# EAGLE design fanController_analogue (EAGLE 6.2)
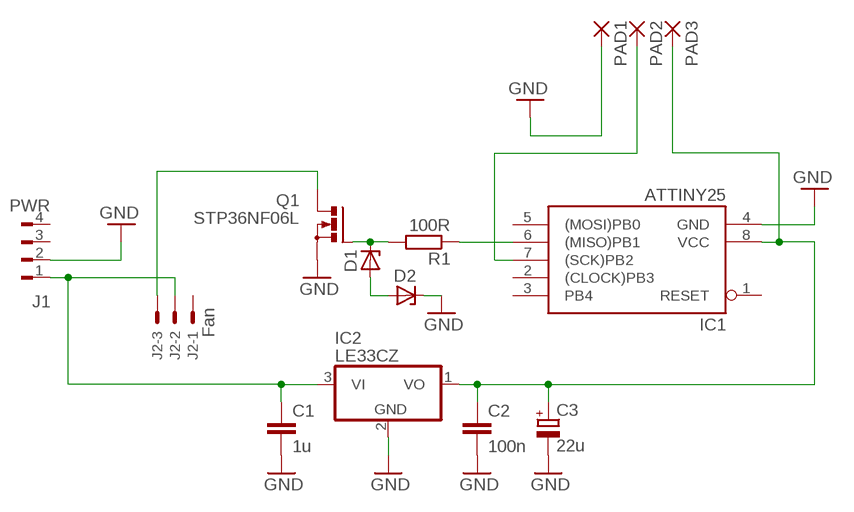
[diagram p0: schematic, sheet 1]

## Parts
C1  1u  C2.5/2  [C2.5-2]
C2  100n  C2.5/2  [C2.5-2]
C3  22u  CPOL-EUE2-4  [E2-4]
D1  ZENER-DIODEZD-5  [ZDIO-5]
D2  ZENER-DIODEZD-5  [ZDIO-5]
IC1  ATTINY25  TINY22P  [DIL08]
IC2  LE33CZ  78L05Z  [TO92]
J1  PWR  FLOP-4W827001  [827001]
J2  Fan  22-23-2031  [22-23-2031]
PAD1  2,54/1,1  [2,54/1,1]
PAD2  2,54/1,1  [2,54/1,1]
PAD3  2,54/1,1  [2,54/1,1]
Q1  STP36NF06L  BUZ11BV  [TO220BV]
R1  100R  R-EU_0207/7  [0207/7]

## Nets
GND: C1.2 C2.2 C3.- D2.C IC1.4(GND) IC2.2(GND) J1.2 PAD1.1(P) Q1.S
N$1: D1.C Q1.G R1.2
N$2: C1.1 IC2.3(VI) J1.1 J2.2
N$3: IC1.7((SCK)PB2) PAD2.1(P)
N$5: D1.A D2.A
N$6: IC1.6((MISO)PB1) R1.1
N$9: J2.3 Q1.D
VCC: C2.1 C3.+ IC1.8(VCC) IC2.1(VO) PAD3.1(P)
Unconnected: IC1.1(RESET) IC1.2((CLOCK)PB3) IC1.3(PB4) IC1.5((MOSI)PB0) J1.3 J1.4 J2.1

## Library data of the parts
C1 C2 = capacitor-wima:C: CAPACITOR
C3 = rcl:CPOL-EU: POLARIZED CAPACITOR, European symbol
D1 D2 = diode:ZENER-DIODE: Z-Diode
IC1 = atmel:TINY22: MICROCONTROLLER 1K ROM 128 bytes RAM 128 bytes EEPROM; OC_FARNELL: unknown; OC_NEWARK: unknown
IC2 = linear:78*: Positive VOLTAGE REGULATOR Source: http://cache.national.com/ds/LM/LM78L05.pdf http://www.fairchildsemi.com/ds/LM/LM7805.pdf
J1 = con-amp:FLOP-4W: MATE N-LOCK Floppy / HDD conector Distributor: Bürklin 71F972
J2 = con-molex:22-23-2031: .100" (2.54mm) Center Header - 3 Pin; MF: MOLEX; MPN: 22-23-2031; OC_FARNELL: 1462950; OC_NEWARK: 30C0862
PAD1-PAD3 = wirepad:2,54/1,1: THROUGH-HOLE PAD
Q1 = transistor-power:BUZ11: N-CHANNEL MOS FET
R1 = resistor:R-EU_: RESISTOR, European symbol

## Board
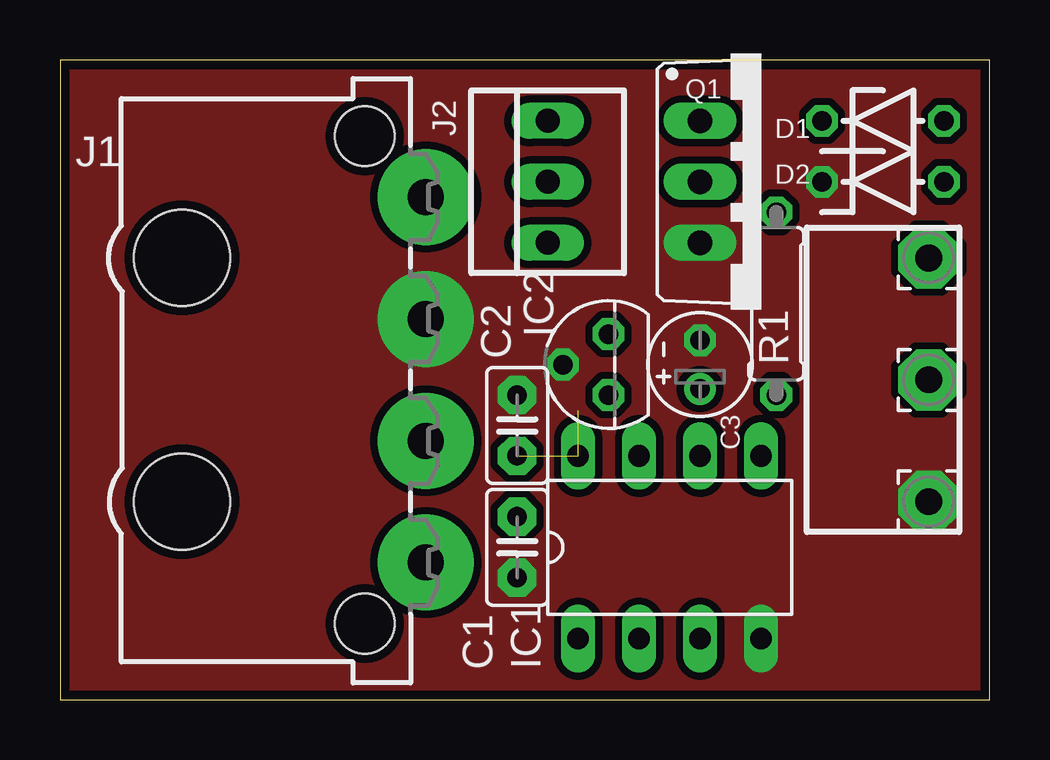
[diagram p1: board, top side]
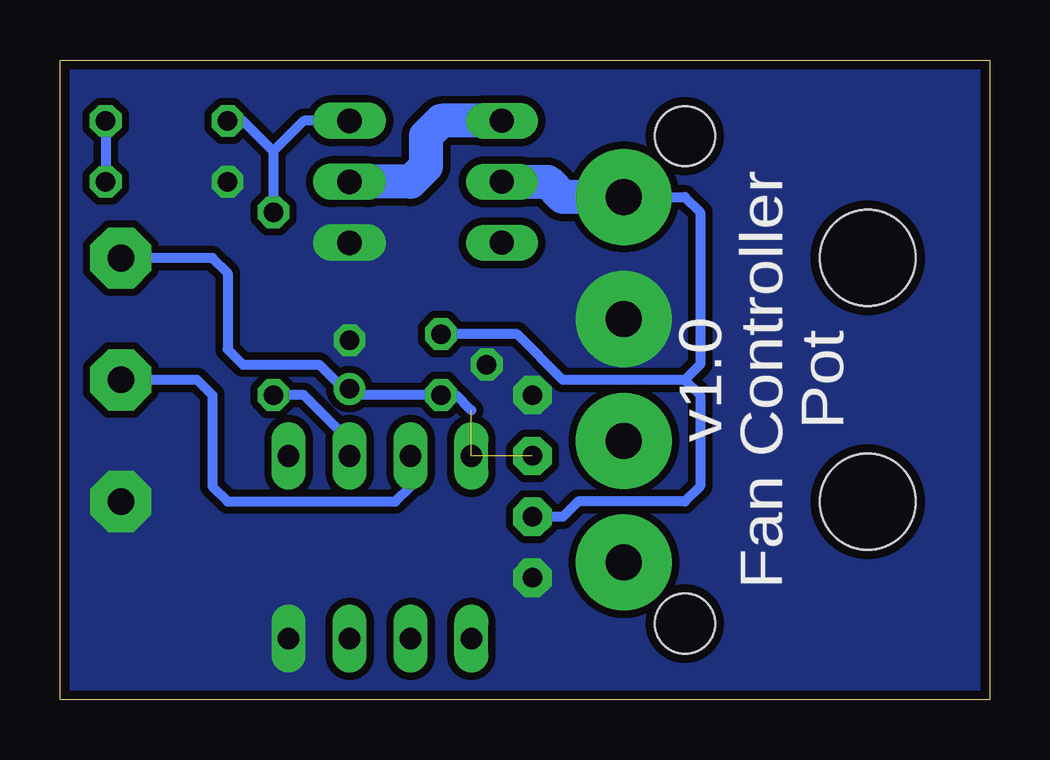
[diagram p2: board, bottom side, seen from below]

Size 38.73 x 26.67 mm. Coordinates in mm from the lower left corner, seen from the top.
Outline: 0,0 38.73,0 38.73,26.67 0,26.67 0,0
Copper layers (1*16): Top 0.0356mm / dielectric 1.5011mm / Bottom 0.0356mm
Design rules: minimum track width 6mil, minimum drill 13mil, track to track 6mil, track to pad 6mil, pad to pad 6mil, via to via 6mil, smd to smd 6mil, copper to edge 15mil, drill to drill 6mil, minimum pad ring 10mil, minimum via ring 7mil, stop-mask expansion 4mil, vias tented up to drill 0mil, thermal gap 10mil

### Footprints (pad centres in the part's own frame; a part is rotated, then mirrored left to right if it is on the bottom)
C2.5-2 = drill 0.813 pad 1.6 octagon: 1 -1.27,0; 2 1.27,0
E2-4 = drill 0.813 pad 1.27: + -1.016,0 | drill 0.813 pad 1.27 octagon: - 1.016,0
ZDIO-5 = drill 0.813 octagon: A 2.54,0; C -2.54,0
DIL08 = drill 0.9 long: 1 -3.81,-3.81; 2 -1.27,-3.81; 3 1.27,-3.81; 4 3.81,-3.81; 5 3.81,3.81; 6 1.27,3.81; 7 -1.27,3.81; 8 -3.81,3.81
TO92 = drill 0.813 octagon: 1 -1.27,0; 2 0,1.905; 3 1.27,0
827001 = drill 1.5 pad 4: 1 -7.62,0; 2 -2.54,0; 3 2.54,0; 4 7.62,0 | hole 4: 5.08,-10.16; -5.08,-10.16 | hole 2.5: 10.16,-2.54; -10.16,-2.54
22-23-2031 = drill 1 long: 1 -2.54,0; 2 0,0; 3 2.54,0
2,54/1,1 = drill 1.118 pad 2.54 octagon: 1 0,0
TO220BV = drill 1.016 long: D 0,-2.54; G -2.54,-2.54; S 2.54,-2.54
0207/7 = drill 0.813 octagon: 1 -3.81,0; 2 3.81,0

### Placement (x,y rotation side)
C1  19.05,6.35 270 top
C2  19.05,11.43 90 top
C3  26.67,13.97 90 top
D1  34.29,24.13 0 top
D2  34.29,21.59 0 top
IC1  25.4,6.35 0 top
IC2  22.86,13.97 90 top
J1  15.24,13.34 270 top
J2  20.32,21.59 90 top
PAD1  36.2,8.26 0 top
PAD2  36.2,13.34 0 top
PAD3  36.2,18.41 0 top
Q1  29.21,21.59 270 top
R1  29.84,16.51 90 top

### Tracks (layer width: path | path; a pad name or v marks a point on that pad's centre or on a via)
GND
  pour Bottom (isolate 0.305, no thermals): 0,26.67 38.73,26.67 38.73,0 0,0
  pour Top (isolate 0.305, no thermals): 0,26.67 38.73,26.67 38.73,0 0,0
N$1
  Bottom 0.406: Q1.G 28.57,24.13 29.84,22.86 | 29.84,22.86 R1.2 | 29.84,22.86 31.11,24.13 D1.C
N$2
  Bottom 0.406: 12.7,13.34 12.06,12.7 12.06,8.89 12.7,8.26 17.14,8.26 17.78,7.62 C1.1 | IC2.3 19.68,15.24 17.78,13.34 12.7,13.34 | J1.1 12.7,20.95 12.06,20.32 12.06,13.97 12.7,13.34
  Bottom 1.422: J1.1 17.78,20.95 18.41,21.59 J2.2
N$3
  Bottom 0.406: IC1.7 24.13,8.89 24.77,8.26 31.75,8.26 32.38,8.89 32.38,12.7 33.02,13.34 PAD2.1
N$5
  Bottom 0.406: D1.A D2.A
N$6
  Bottom 0.406: IC1.6 26.67,10.79 28.57,12.7 R1.1
N$9
  Bottom 1.422: J2.3 22.86,24.13 23.5,23.5 23.5,22.23 24.13,21.59 Q1.D
VCC  (2 unrouted)
  Bottom 0.406: 26.67,12.7 IC2.1 22.23,12.7 21.59,12.06 | 26.67,12.7 C3.+ | 26.67,12.7 27.94,13.97 31.11,13.97 31.75,14.61 31.75,17.78 32.38,18.41 PAD3.1

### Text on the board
bNames: Pot | Fan Controller | v1.0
